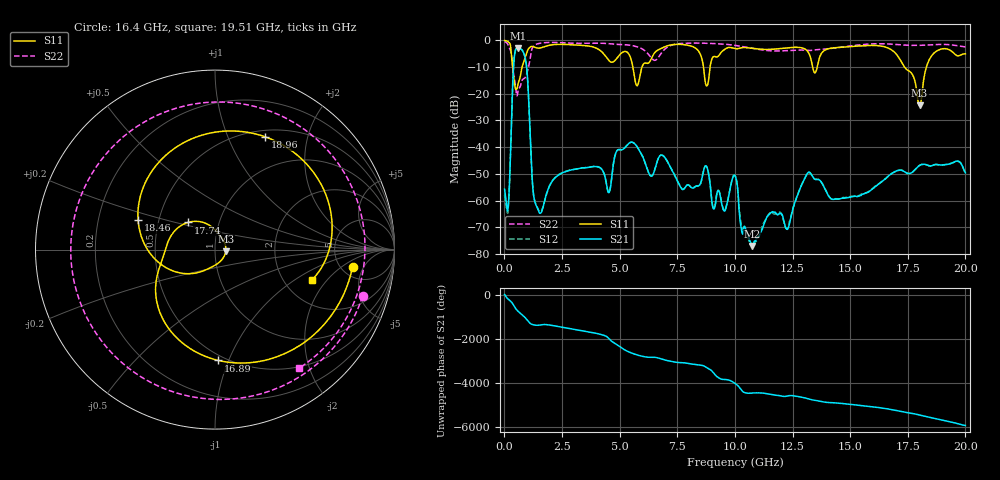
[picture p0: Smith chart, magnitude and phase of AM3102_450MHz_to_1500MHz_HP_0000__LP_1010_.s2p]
!Agilent Technologies,E8364B,MY43040894,A.07.50.67
!Agilent E8364B: A.07.50.67
!Date: Thursday, January 11, 2018 05:17:11
!Correction: S11(Full 2 Port(1,2))
!S21(Full 2 Port(1,2))
!S12(Full 2 Port(1,2))
!S22(Full 2 Port(1,2))
!S2P File: Measurements: S11, S21, S12, S22:
# Hz S  dB  R 50
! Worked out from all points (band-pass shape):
!   1601 points, 10 MHz to 20 GHz, reference 50 ohm
!   highest |S21| = -2.86 dB at 584.7 MHz (marker M1); lowest = -76.9 dB at 10.74 GHz (marker M2)
!   |S21| within 3 dB of the highest: 435.3 MHz to 882.2 MHz (446.8 MHz wide, 67.8 % of centre)
!   lowest |S11| = -24.3 dB at 18.01 GHz (marker M3), VSWR 1.13, Z = 56.4 - j1.07 ohm
!   |S11| at or under -10 dB: 356.7 MHz to 768.7 MHz (412.1 MHz wide, 73.2 % of centre); 5.574 GHz to 5.971 GHz (396.3 MHz wide, 6.86 % of centre); 17.36 GHz to 18.31 GHz (953 MHz wide, 5.34 % of centre)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
!   |S22| runs from -20.8 to -0.5 dB; largest |S21 - S12| = 0.0034
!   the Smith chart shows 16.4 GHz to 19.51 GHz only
!   S11 on the Smith chart (normalised r, x): 16.4 GHz: 6.26, -3.06; 16.89 GHz: 0.46, -0.92; 17.74 GHz: 0.71, +0.23; 18.46 GHz: 0.38, +0.16; 18.96 GHz: 0.58, +1.38; 19.51 GHz: 2.84, -1.40
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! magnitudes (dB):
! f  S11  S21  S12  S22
! 10 MHz  -0.1  -55.7  -57.9  -0.5
! 172.4 MHz  -0.6  -61.5  -62.1  -1.9
! 409.8 MHz  -14.4  -8.4  -8.4  -13.2
! 584.7 MHz  -16.6  -2.9  -2.9  -19.3
! 934.5 MHz  -5.5  -7.9  -7.9  -13.3
! 1.247 GHz  -2.4  -56.4  -56.3  -2.3
! 1.459 GHz  -2.9  -63.2  -63.2  -1.3
! 3.346 GHz  -1.9  -47.8  -47.8  -1.1
! 5.757 GHz  -17.0  -39.8  -39.8  -2.4
! 6.682 GHz  -3.5  -44.1  -44.1  -6.4
! 10.01 GHz  -3.1  -50.7  -50.7  -1.9
! 10.74 GHz  -3.0  -76.9  -76.6  -3.0
! 13.34 GHz  -8.6  -50.5  -50.6  -3.7
! 16.4 GHz  -2.2  -52.7  -52.7  -1.3
! 16.68 GHz  -3.0  -50.7  -50.7  -1.4
! 16.89 GHz  -4.2  -49.4  -49.4  -1.5
! 17.74 GHz  -13.4  -49.1  -49.1  -1.9
! 18.01 GHz  -24.3  -46.8  -46.8  -1.9
! 18.46 GHz  -6.8  -47.0  -47.1  -1.7
! 18.96 GHz  -3.3  -46.7  -46.6  -1.5
! 19.51 GHz  -4.9  -45.5  -45.6  -1.8
! 20 GHz  -5.0  -49.6  -49.7  -2.4
